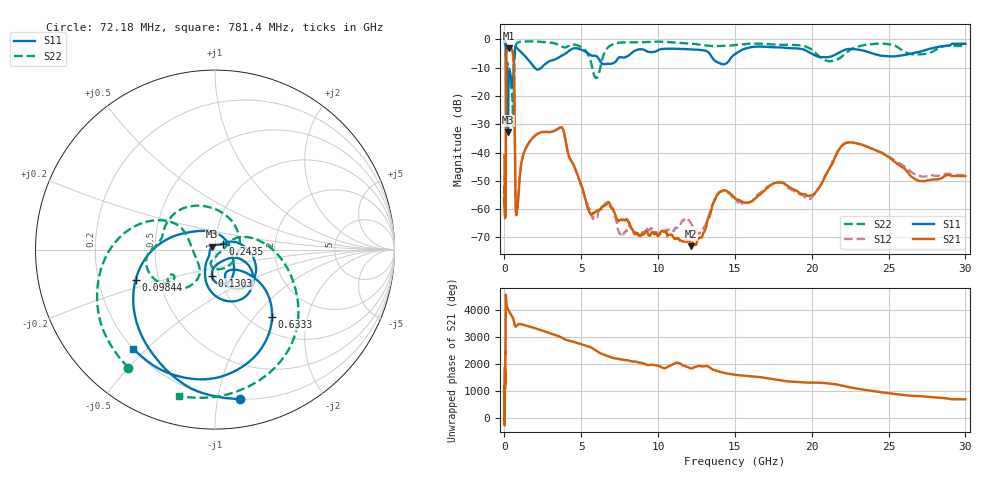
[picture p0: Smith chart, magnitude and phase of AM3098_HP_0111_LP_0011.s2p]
! Date/Time: Thu, Feb 28, 2019 8:38 AM
! Network Analyzer: Agilent Technologies E8364B Rev: A.07.50.67
! Sweep from 0.010 to 30.000 GHz, 1601 Points, Sweep Type: LOG
! Power Supply: 5.023 V, 0.002 A
# Hz S DB R 50
!freq MagS11 AngS11 MagS21 AngS21 MagS12 AngS12 MagS22 AngS22
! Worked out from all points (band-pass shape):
!   1601 points, 10 MHz to 30 GHz, reference 50 ohm
!   highest |S21| = -3.09 dB at 267.8 MHz (marker M1); lowest = -73.1 dB at 12.13 GHz (marker M2)
!   |S21| within 3 dB of the highest: 120.9 MHz to 577.3 MHz (456.4 MHz wide, 131 % of centre)
!   lowest |S11| = -32.8 dB at 231.6 MHz (marker M3), VSWR 1.05, Z = 48.5 + j1.63 ohm
!   |S11| at or under -10 dB: 102.2 MHz to 598.6 MHz (496.4 MHz wide, 142 % of centre); 1.974 GHz to 2.4 GHz (425.9 MHz wide, 19.5 % of centre)
!   |S22| runs from -30.7 to -0.5 dB; largest |S21 - S12| = 0.014
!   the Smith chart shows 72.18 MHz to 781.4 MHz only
!   S11 on the Smith chart (normalised r, x): 72.18 MHz: 0.20, -1.16; 98.44 MHz: 0.37, -0.16; 130.3 MHz: 0.93, -0.28; 243.5 MHz: 1.09, +0.07; 633.3 MHz: 1.25, -1.24; 781.4 MHz: 0.20, -0.46
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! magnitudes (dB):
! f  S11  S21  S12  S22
! 10 MHz  -0.4  -41.5  -42.3  -0.5
! 38.04 MHz  -0.5  -60.1  -58.1  -0.8
! 72.18 MHz  -1.5  -54.1  -55.4  -1.8
! 85.57 MHz  -2.6  -53.4  -55.5  -2.8
! 98.44 MHz  -6.5  -27.3  -27.2  -7.3
! 130.3 MHz  -16.6  -5.1  -5.0  -10.2
! 144.7 MHz  -20.1  -4.1  -4.1  -11.3
! 186.8 MHz  -11.0  -3.7  -3.7  -8.1
! 231.6 MHz  -32.8  -3.2  -3.2  -9.8
! 243.5 MHz  -25.2  -3.2  -3.1  -10.1
! 267.8 MHz  -15.6  -3.1  -3.1  -10.4
! 550.5 MHz  -15.9  -5.0  -4.9  -27.1
! 633.3 MHz  -6.2  -13.6  -13.5  -12.1
! 721.3 MHz  -2.7  -56.2  -56.8  -2.3
! 781.4 MHz  -2.9  -61.8  -60.4  -1.5
! 2.084 GHz  -10.5  -33.6  -33.6  -0.7
! 3.742 GHz  -5.7  -31.2  -31.1  -2.5
! 5.556 GHz  -5.3  -61.3  -60.0  -6.7
! 7.926 GHz  -6.2  -63.5  -67.4  -1.0
! 12.13 GHz  -3.5  -73.1  -64.9  -1.5
! 22.56 GHz  -3.4  -36.4  -36.4  -3.5
! 30 GHz  -1.5  -48.3  -47.9  -2.3
